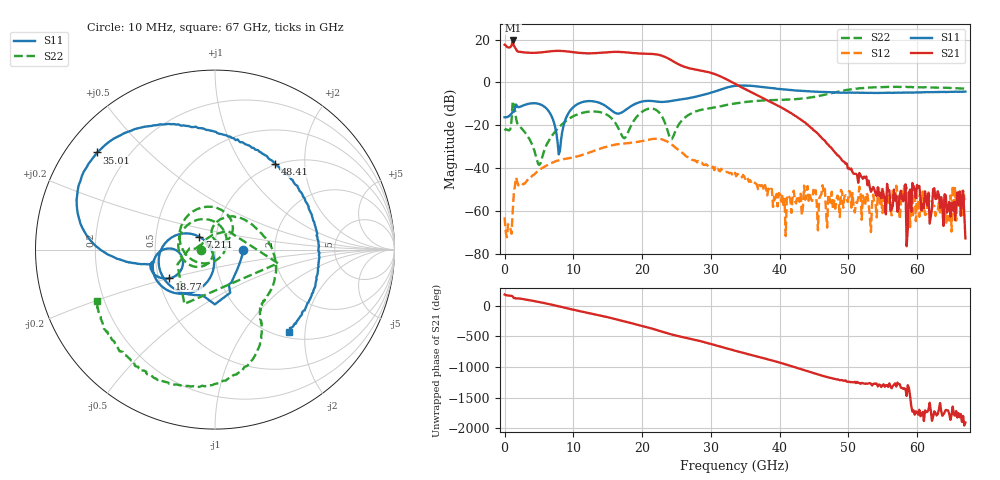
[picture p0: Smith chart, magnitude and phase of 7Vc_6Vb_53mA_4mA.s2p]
! MARKI MICROWAVE INC.
! Date:  05/05/2020
! Model Number:  APM-7099CH
! Description:  2-port Small Signal S-parameter data for APM-7099CH
! Frequency Range:  10 MHz to 67 GHz
! Port Configuration:  PORT 1: Input
!  PORT 2: Output
! Bias Condition: Vc = +7V, Vb = +6V
! APM-7099CH s2p files are only valid for small signal conditions (below -5 dBm input power)
!S2P File: Measurements: Mag<S11> Ang<S11>, Mag<S21> Ang<S21>, Mag<S12> Ang<S12>, Mag<S22> Ang<S22>!row 1
# Hz S  dB  R 50
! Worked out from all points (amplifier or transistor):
!   401 points, 10 MHz to 67 GHz, reference 50 ohm
!   highest |S21| = 19.6 dB at 1.182 GHz (marker M1)
!   |S21| within 3 dB of that: start of sweep to 352.4 MHz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
!   unconditionally stable (mu >= 1): start of sweep to end of sweep
!   at 11.06 GHz: K = 4.49, MAG = 14.5 dB, |S12| = -34.1 dB
!   at 33.51 GHz: K = 18.98, MAG = 5.0 dB, |S12| = -42.2 dB
!   at 67 GHz: K = 355636.68, MAG = -67.6 dB, |S12| = -54.6 dB
!   S11 on the Smith chart (normalised r, x): 10 MHz: 1.36, -0.01; 7.211 GHz: 0.83, +0.12; 18.77 GHz: 0.57, -0.20; 35.01 GHz: 0.09, +0.36; 48.41 GHz: 0.98, +1.43; 67 GHz: 1.11, -1.64
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1e7  -16.25 -0.7  17.64 178.7  -63.03 46.4  -22.46 -176.8
1.182325e9  -13.76 -63.5  19.64 148.0  -60.55 71.0  -8.89 -12.2
1.68475e9  -10.31 -90.2  15.62 114.5  -44.37 -80.0  -16.96 177.5
4.531825e9  -9.72 -161.7  13.89 67.4  -42.31 -166.5  -34.13 147.5
7.211425e9  -18.99 140.6  14.73 4.0  -37.14 129.9  -23.54 -112.4
9.221125e9  -14.74 -103.2  14.47 -49.8  -35.44 86.2  -17.27 -135.1
1.123082e10  -9.23 -138.2  13.75 -98.8  -33.90 50.0  -14.25 -170.1
1.3408e10  -9.11 -168.6  13.77 -149.7  -31.47 8.7  -13.63 145.3
1.508275e10  -11.86 178.6  14.20 166.9  -29.76 -28.8  -15.45 100.7
1.709245e10  -13.92 -153.5  14.21 109.6  -28.61 -77.3  -24.99 -3.4
1.87672e10  -10.36 -148.1  13.75 62.1  -28.03 -116.9  -18.00 -147.6
2.07769e10  -8.58 -162.3  13.40 4.3  -26.79 -166.9  -12.41 133.4
2.245165e10  -9.03 -168.8  12.89 -50.7  -26.34 139.5  -13.92 67.4
2.41264e10  -8.69 -167.3  10.63 -107.2  -28.59 82.5  -26.36 60.5
2.580115e10  -7.88 -168.5  7.76 -152.0  -32.78 41.1  -17.70 94.2
2.94856e10  -5.28 -174.5  4.96 108.9  -38.68 -10.4  -12.24 36.4
3.3505e10  -1.58 156.6  -0.57 -16.8  -42.21 -65.7  -9.79 -1.3
3.501228e10  -1.40 140.5  -3.12 -60.8  -45.10 -83.3  -9.12 -14.2
4.472582e10  -4.19 75.8  -21.46 -14.7  -55.37 29.0  -6.89 -55.9
4.841028e10  -4.67 55.0  -34.08 -122.9  -52.84 -55.4  -4.34 -66.9
5.594665e10  -4.80 9.4  -50.37 171.6  -51.59 -141.7  -2.10 -109.3
6.7e10  -4.22 -48.2  -72.85 -106.2  -54.65 0.2  -2.87 -156.3
